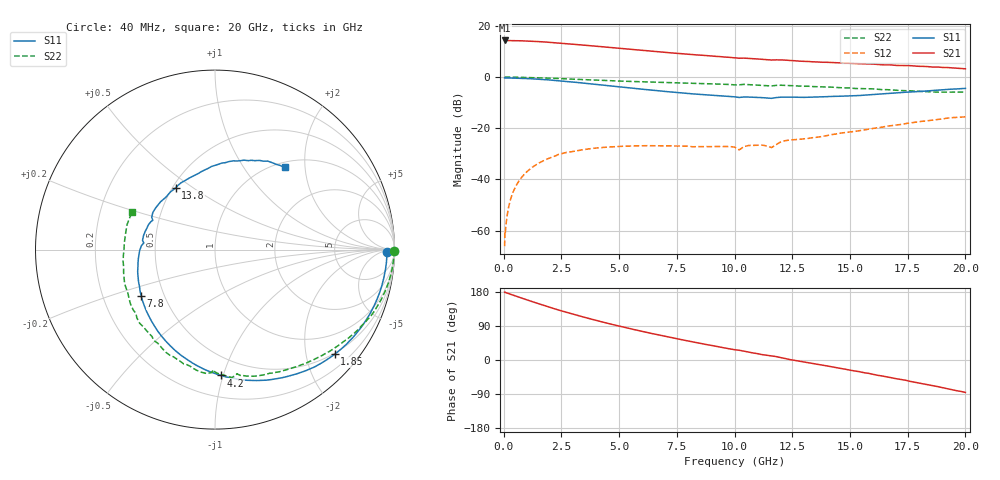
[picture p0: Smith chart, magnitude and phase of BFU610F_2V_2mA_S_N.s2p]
! Filename:  P:\Prog\Test\Noise\ATS_data\Testdata_Net\SplitFiles\BFU610_2W_A5_HighFreq_2V_2mA_D.s2p
! Date/Time: Wed 10/Aug/2011 16:55:49
! BFU610_2W_A5_HighFreq_2V_1mA_10mA_Bias2_R.s2p
! MDIF S-parameter v. bias file
! BFU610_2W_A5_HighFreq_2V_1mA_10mA
! Date/time Mon Aug 08 14:20:39 2011
! VAR V_out= 2.0002
! VAR I_out= 1.9950
! VAR V_in= 0.8693
! VAR I_in= 0.0151
! Device data file deembeded for feedlines and parallel
! Original file: \SplitFiles\BFU610_2W_A5_HighFreq_2V_2mA_R.s2p
! Feed-files: PR003V01_101208_Feed1.s2p, PR003V01_101208_Feed2.s2p
! Parallel-file: PR003V01_101208_Par.s2p
# MHz S MA R 50
!  Freq-MHz  S11-mag  S11-arg  S21-mag  S21-arg  S12-mag  S12-arg  S22-mag  S22-arg
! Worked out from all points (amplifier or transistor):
!   167 points, 40 MHz to 20 GHz, reference 50 ohm
!   highest |S21| = 14.3 dB at 40 MHz (marker M1)
!   |S21| within 3 dB of that: start of sweep to 4.909 GHz
!   unconditionally stable (mu >= 1): 6.656 GHz to 19.07 GHz
!   at 550 MHz: K = 0.01, MSG = 28.3 dB, |S12| = -42.3 dB
!   at 4.2 GHz: K = 0.54, MSG = 19.7 dB, |S12| = -27.6 dB
!   at 20 GHz: K = 0.94, MSG = 9.4 dB, |S12| = -15.6 dB
!   lowest NFmin = 0.92 dB at 400 MHz
!   S11 on the Smith chart (normalised r, x): 40 MHz: 41, -15; 1.85 GHz: 0.48, -2.59; 4.2 GHz: 0.36, -0.99; 7.8 GHz: 0.37, -0.25; 13.8 GHz: 0.52, +0.43; 20 GHz: 1.09, +1.57
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40  0.9582 -0.9  5.186 179.0  0.000494 84.4  0.9961 -0.3
50  0.9502 -1.3  5.165 179.1  0.0008121 120.9  0.9963 -0.5
60  0.9582 -1.1  5.18 178.2  0.0009315 94.6  0.9971 -0.6
180  0.9579 -4.1  5.154 176.1  0.002382 90.6  0.9968 -1.9
460  0.9529 -10.5  5.149 170.1  0.006385 86.5  0.9942 -5.0
1150  0.9267 -26.0  5.033 155.8  0.01605 74.5  0.9795 -12.4
1850  0.8861 -41.2  4.816 141.9  0.02461 63.6  0.957 -19.5
2700  0.8199 -58.7  4.507 126.2  0.03343 51.4  0.9201 -27.4
3400  0.7657 -72.3  4.224 114.2  0.03775 43.7  0.8926 -33.4
4200  0.7023 -87.2  3.929 101.4  0.04166 35.8  0.8618 -39.6
5400  0.6169 -108.2  3.508 83.7  0.0447 26.7  0.8228 -48.4
6800  0.5325 -131.7  3.082 65.0  0.0453 19.2  0.7833 -58.1
7800  0.4856 -148.0  2.836 52.5  0.04484 16.6  0.7599 -64.9
9400  0.4298 -173.4  2.502 33.7  0.04377 17.0  0.7258 -76.1
10200  0.3984 174.7  2.329 25.7  0.03767 18.9  0.7034 -79.9
11600  0.3832 154.7  2.15 10.7  0.04178 27.7  0.669 -90.8
12000  0.4035 149.2  2.162 6.3  0.05398 35.5  0.6916 -94.1
13400  0.4062 127.5  1.983 -9.3  0.06527 29.2  0.6506 -107.6
13800  0.4086 122.3  1.945 -13.4  0.06896 29.5  0.6403 -111.2
16800  0.4835 85.5  1.725 -46.9  0.1124 16.9  0.5604 -147.0
18400  0.5371 67.9  1.594 -65.9  0.1408 4.0  0.5162 -172.7
20000  0.6003 49.8  1.449 -85.5  0.1669 -12.7  0.5075 155.3
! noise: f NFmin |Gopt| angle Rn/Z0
400  0.9204  0.7033  3.708  0.5803
700  0.9485  0.6863  7.165  0.584
1150  0.9909  0.664  12.26  0.5859
1600  1.034  0.6449  17.23  0.5836
2050  1.077  0.628  22.05  0.5775
2600  1.13  0.6093  27.74  0.5653
3500  1.218  0.5805  36.71  0.5355
4400  1.308  0.5512  45.54  0.4957
5600  1.429  0.5099  57.92  0.4312
8000  1.681  0.4465  89.83  0.2856
